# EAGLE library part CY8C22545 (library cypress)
PSoC® Programmable System-on-Chip TM M8C Processor Speeds up to 24 MHz Source: http://www.cypress.com .. CY8C213452.pdf
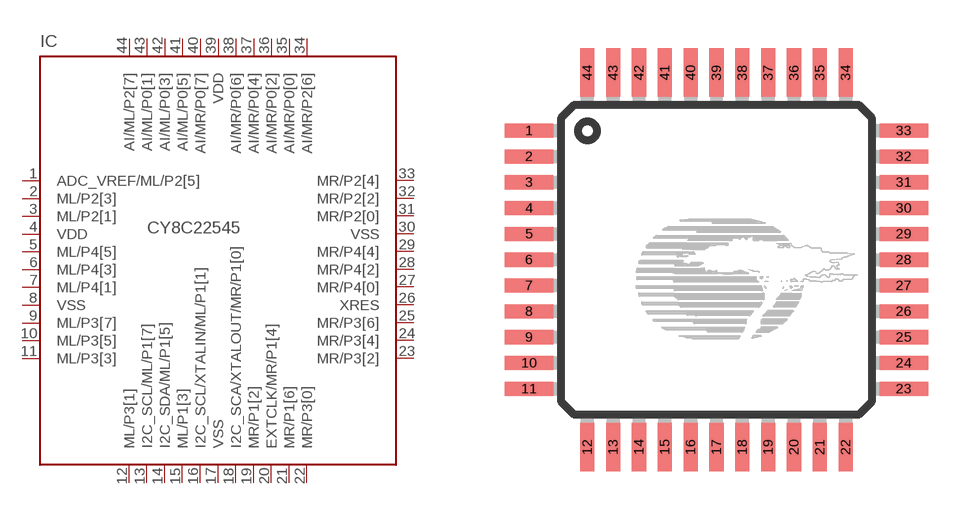
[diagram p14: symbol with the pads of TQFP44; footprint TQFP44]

Designator prefix IC

## CY8C22545T (OC_FARNELL: unknown; OC_NEWARK: unknown)  [TQFP44]
1  ADC_VREF/ML/P2[5]
2  ML/P2[3]
3  ML/P2[1]
4  VDD  pwr
5  ML/P4[5]
6  ML/P4[3]
7  ML/P4[1]
8  VSS  pwr
9  ML/P3[7]
10  ML/P3[5]
11  ML/P3[3]
12  ML/P3[1]
13  I2C_SCL/ML/P1[7]
14  I2C_SDA/ML/P1[5]
15  ML/P1[3]
16  I2C_SCL/XTALIN/ML/P1[1]
17  VSS  pwr
18  I2C_SCA/XTALOUT/MR/P1[0]
19  MR/P1[2]
20  EXTCLK/MR/P1[4]
21  MR/P1[6]
22  MR/P3[0]
23  MR/P3[2]
24  MR/P3[4]
25  MR/P3[6]
26  XRES  in
27  MR/P4[0]
28  MR/P4[2]
29  MR/P4[4]
30  VSS  pwr
31  MR/P2[0]
32  MR/P2[2]
33  MR/P2[4]
34  AI/MR/P2[6]
35  AI/MR/P0[0]
36  AI/MR/P0[2]
37  AI/MR/P0[4]
38  AI/MR/P0[6]
39  VDD  pwr
40  AI/MR/P0[7]
41  AI/ML/P0[5]
42  AI/ML/P0[3]
43  AI/ML/P0[1]
44  AI/ML/P2[7]

## Footprint TQFP44 (pad centres in mm)
44-Pin TQFP Source: http://www.cypress.com .. CY8C213452.pdf
smd 1.5 x 0.44: 1 -5.8,4; 2 -5.8,3.2; 3 -5.8,2.4; 4 -5.8,1.6; 5 -5.8,0.8; 6 -5.8,0; 7 -5.8,-0.8; 8 -5.8,-1.6; 9 -5.8,-2.4; 10 -5.8,-3.2; 11 -5.8,-4; 23 5.8,-4; 24 5.8,-3.2; 25 5.8,-2.4; 26 5.8,-1.6; 27 5.8,-0.8; 28 5.8,0; 29 5.8,0.8; 30 5.8,1.6; 31 5.8,2.4; 32 5.8,3.2; 33 5.8,4
smd 0.44 x 1.5: 12 -4,-5.8; 13 -3.2,-5.8; 14 -2.4,-5.8; 15 -1.6,-5.8; 16 -0.8,-5.8; 17 0,-5.8; 18 0.8,-5.8; 19 1.6,-5.8; 20 2.4,-5.8; 21 3.2,-5.8; 22 4,-5.8; 34 4,5.8; 35 3.2,5.8; 36 2.4,5.8; 37 1.6,5.8; 38 0.8,5.8; 39 0,5.8; 40 -0.8,5.8; 41 -1.6,5.8; 42 -2.4,5.8; 43 -3.2,5.8; 44 -4,5.8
